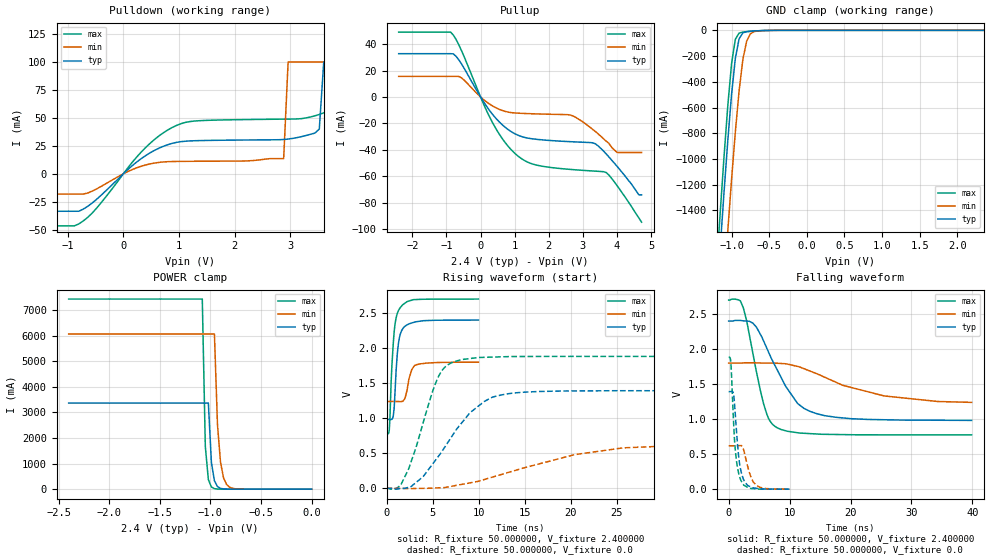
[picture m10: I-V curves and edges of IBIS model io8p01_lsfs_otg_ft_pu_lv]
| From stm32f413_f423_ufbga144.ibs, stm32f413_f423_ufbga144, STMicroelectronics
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|   Model io8p01_lsfs_otg_ft_pu_lv
[Model]  io8p01_lsfs_otg_ft_pu_lv
Model_type I/O
Polarity   Non-Inverting
Enable   Active-Low
Vinl =   0.720000V
Vinh =   1.680000V
Vmeas =  1.200000V
Cref =   50.000000pF
Rref =   100.000000M
Vref =   0.0V
C_comp   7.971100pF   7.737700pF   8.264100pF
[Temperature Range]   25.000000   0.125000k   -40.000000
[Pullup Reference]   2.400000V   1.800000V   2.700000V
[Pulldown Reference]   0.0V   0.0V   0.0V
[POWER Clamp Reference]   2.400000V   1.800000V   2.700000V
[GND Clamp Reference]   0.0V   0.0V   0.0V
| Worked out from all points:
|   slope of the pulldown table from 0 to 0.36 V, typ, clamps not added: 24.1 ohm
|   slope of the pullup table from 0 to 0.36 V, typ, clamps not added: 26.8 ohm
|   GND clamp passes 1 mA (typ) near -0.52 V on its own axis
|   POWER clamp passes 1 mA (typ) near -0.81 V on its own axis
|   rising waveform, R_fixture 50.000000, V_fixture 2.400000: 20-80 % time 477ps typ, 591ps min, 489ps max; typ from 0.983 V to 2.4 V
|   rising waveform, R_fixture 50.000000, V_fixture 0.0: 20-80 % time 4.79ns typ, 10.6ns min, 2.68ns max; typ from 0.001 V to 1.39 V
|   falling waveform, R_fixture 50.000000, V_fixture 2.400000: 20-80 % time 5.25ns typ, 11.3ns min, 2.79ns max; typ from 2.4 V to 0.983 V
|   falling waveform, R_fixture 50.000000, V_fixture 0.0: 20-80 % time 916ps typ, 1.27ns min, 800ps max; typ from 1.39 V to 0.001 V
[Pulldown]
|Voltage   I(typ)   I(min)   I(max)
-2.4V     -33.44mA   -18.11mA   -46.51mA
-800mV    -33.44mA   -18.11mA   -44.78mA
1.04V     28.81mA    11.14mA    44.91mA
2.88V     30.7mA     13.62mA    48.89mA
2.96V     31.1mA     100mA      48.94mA
3.52V     40mA       100mA      53.06mA
3.6V      100mA      100mA      54.54mA
3.92V     100mA      100mA      60mA
4V        100mA      100mA      100mA
4.4V      100mA      100mA      100mA
4.48V     100mA      100mA      1A
4.8V      100mA      100mA      1A
[Pullup]
|Voltage   I(typ)   I(min)   I(max)
-2.4V     32.71mA    15.53mA    49.05mA
-880mV    32.71mA    15.53mA    49.05mA
-560mV    25.05mA    14.45mA    35.12mA
320mV     -12.14mA   -6.322mA   -17.91mA
960mV     -27.18mA   -12mA      -41.54mA
1.52V     -31.65mA   -12.71mA   -50.67mA
2.64V     -33.82mA   -13.73mA   -54.81mA
3.28V     -34.63mA   -24.4mA    -55.96mA
3.68V     -43mA      -33.4mA    -57.12mA
4V        -52.4mA    -42mA      -67mA
4.64V     -74mA      -42mA      -91.5mA
4.72V     -74mA      -42mA      -94.7mA
[GND_clamp]
|Voltage   I(typ)   I(min)   I(max)
-2.4V     -9.766A    -9.942A    -9.572A
-1.2V     -2.124A    -2.851A    -1.855A
-1.15V    -1.682A    -2.408A    -1.408A
-1.1V     -1.256A    -1.975A    -979.8mA
-1.05V    -854.9mA   -1.556A    -584.5mA
-1V       -496.5mA   -1.158A    -257.5mA
-950mV    -217.7mA   -789.6mA   -69.52mA
-900mV    -65.57mA   -469.8mA   -21.5mA
-850mV    -19.64mA   -226.4mA   -13.56mA
-800mV    -9.753mA   -84.21mA   -10.47mA
-700mV    -4.923mA   -9.884mA   -5.807mA
2.35V     0A         0A         0A
[POWER_clamp]
|Voltage   I(typ)   I(min)   I(max)
-2.4V     3.365A     6.064A     7.43A
-1.08V    3.365A     6.064A     7.43A
-1.05V    3.365A     6.064A     1.669A
-1.02V    3.365A     6.064A     375.2mA
-990mV    1.047A     6.064A     84.45mA
-960mV    325.8mA    6.064A     19.12mA
-930mV    101.4mA    2.529A     4.431mA
-900mV    31.63mA    1.055A     1.12mA
-870mV    9.908mA    440.1mA    365.5uA
-840mV    3.145mA    183.6mA    185.6uA
-720mV    90.15uA    5.596mA    88.88uA
0V        0A         0A         0A
[Ramp]
| variable   typ   min   max
dV/dt_r  0.83553/4.78602n   0.37009/10.64511n   1.12843/2.68038n
dV/dt_f  0.85040/5.24450n   0.32604/11.51193n   1.15438/2.78707n
R_load = 50.000000
[Rising Waveform]
R_fixture= 50.000000
V_fixture= 2.400000
V_fixture_min= 1.800000
V_fixture_max= 2.700000
|time   V(typ)   V(min)   V(max)
0s        982.7mV    1.24V      775.9mV
300.3ps   982.4mV    1.24V      838.5mV
520.5ps   983.7mV    1.24V      1.577V
720.7ps   1.023V     1.24V      2.043V
900.9ps   1.324V     1.24V      2.318V
1.161ns   1.905V     1.239V     2.491V
1.401ns   2.151V     1.238V     2.56V
2.002ns   2.312V     1.283V     2.642V
3.043ns   2.371V     1.752V     2.692V
9.97ns    2.4V       1.8V       2.7V
[Rising Waveform]
R_fixture= 50.000000
V_fixture= 0.0
V_fixture_min= 0.0
V_fixture_max= 0.0
|time   V(typ)   V(min)   V(max)
0s        869.3uV    837.3uV    975.6uV
1.602ns   -2.493mV   871uV      62.8mV
2.402ns   14.39mV    -5.665mV   278.6mV
3.924ns   162.3mV    491.7uV    914.2mV
5.526ns   439.4mV    7.08mV     1.565V
7.207ns   765.8mV    33.67mV    1.801V
10.57ns   1.237V     125.2mV    1.869V
13.21ns   1.35V      227.4mV    1.879V
25.63ns   1.393V     577.6mV    1.882V
39.88ns   1.393V     619.1mV    1.882V
[Falling Waveform]
R_fixture= 50.000000
V_fixture= 2.400000
V_fixture_min= 1.800000
V_fixture_max= 2.700000
|time   V(typ)   V(min)   V(max)
0s        2.4V       1.8V       2.7V
2.402ns   2.404V     1.803V     2.59V
4.004ns   2.367V     1.805V     1.926V
5.766ns   2.11V      1.801V     1.209V
6.567ns   1.952V     1.8V       1.006V
7.848ns   1.724V     1.799V     883.1mV
11.29ns   1.227V     1.753V     806.5mV
14.41ns   1.079V     1.65V      788.4mV
25.55ns   991.6mV    1.331V     776.5mV
39.88ns   982.7mV    1.24V      775.9mV
[Falling Waveform]
R_fixture= 50.000000
V_fixture= 0.0
V_fixture_min= 0.0
V_fixture_max= 0.0
|time   V(typ)   V(min)   V(max)
0s        1.393V     619.1mV    1.882V
360.4ps   1.394V     619.1mV    1.804V
840.8ps   1.331V     619mV      890.9mV
1.281ns   832mV      618.6mV    407mV
1.622ns   481.5mV    620.3mV    234.5mV
2.002ns   264.6mV    623mV      126.3mV
2.743ns   91.08mV    460.6mV    45.06mV
3.684ns   29.61mV    166.8mV    10.74mV
4.484ns   14.4mV     58.79mV    5.414mV
9.97ns    869.3uV    837.3uV    975.6uV
